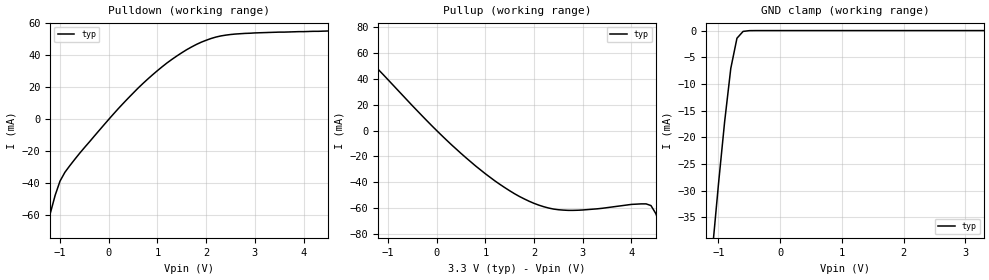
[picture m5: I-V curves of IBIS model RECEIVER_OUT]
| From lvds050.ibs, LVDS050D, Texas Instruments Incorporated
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|   with 100ohm line-to-line and a 10pF cap from each
|   line-to-ground.
|   Receiver Output  MODEL
[Model]   RECEIVER_OUT
Model_type   3-state
| Signals   1R,2R
Vmeas = 1.5V   |Reference voltage for timing measurements
Cref = 8pF   |Timing specification test load capacitance value
Vref = 0   |Timing specification test load voltage; GND
| variable   typ   min   max
C_comp   1.0pF   NA   NA
|   typ   min   max
[Temperature Range]   25.0   NA   NA
[Voltage range]   3.3V   3.0V   3.6V
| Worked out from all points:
|   slope of the pulldown table from 0 to 0.495 V, typ, clamps not added: 30.5 ohm
|   slope of the pullup table from 0 to 0.495 V, typ, clamps not added: 28.4 ohm
|   GND clamp passes 1 mA (typ) near -0.67 V on its own axis
[Pulldown]
|   Voltage   I(typ)   I(min)   I(max)
-3.3V     -346mA     NA         NA
-1.3V     -71mA      NA         NA
-1.1V     -47.5mA    NA         NA
-1V       -38.6mA    NA         NA
-900mV    -33.1mA    NA         NA
-600mV    -21.3mA    NA         NA
200mV     6.84mA     NA         NA
800mV     25.2mA     NA         NA
1.3V      37.6mA     NA         NA
1.9V      48.3mA     NA         NA
2.6V      53.4mA     NA         NA
6.6V      57.7mA     NA         NA
[Pullup]
|   Voltage   I(typ)   I(min)   I(max)
| Note that the[Pullup]voltage table is referenced to Vcc
| and is calculated using Vtable=Vcc - Vmeasured.
-3.3V     130mA      NA         NA
-2V       78.9mA     NA         NA
300mV     -10.8mA    NA         NA
1.2V      -38.9mA    NA         NA
1.9V      -54.5mA    NA         NA
2.3V      -59.7mA    NA         NA
2.7V      -61.5mA    NA         NA
4.3V      -56.5mA    NA         NA
4.4V      -57.8mA    NA         NA
4.6V      -74.1mA    NA         NA
4.7V      -85.9mA    NA         NA
6.6V      -346mA     NA         NA
[GND_clamp]
|   Voltage   I(typ)   I(min)   I(max)
| Outputs in High Impedance (off)
-3.3V     -347mA     NA         NA
-1.1V     -41.4mA    NA         NA
-1V       -28.8mA    NA         NA
-900mV    -17.1mA    NA         NA
-800mV    -7.08mA    NA         NA
-700mV    -1.43mA    NA         NA
-600mV    -153uA     NA         NA
-400mV    -866nA     NA         NA
3.3V      -59.7pA    NA         NA
[POWER_clamp]
|   Voltage   I(typ)   I(min)   I(max)
| Note that the [POWER_clamp] voltage table is referenced to Vcc
| and is calculated using Vtable = Vcc - Vmeasured.
| Outputs in Tri-state.
-3.3V     0A         NA         NA
0V        0A         NA         NA
[Ramp]
| Note: Ramp rate measured on single-ended Output.
|   typ   min   max
dV/dt_r   1.74/700ps   NA   NA
dV/dt_f   1.74/900ps   NA   NA
R_load = 1MOhm   | Represents an open
